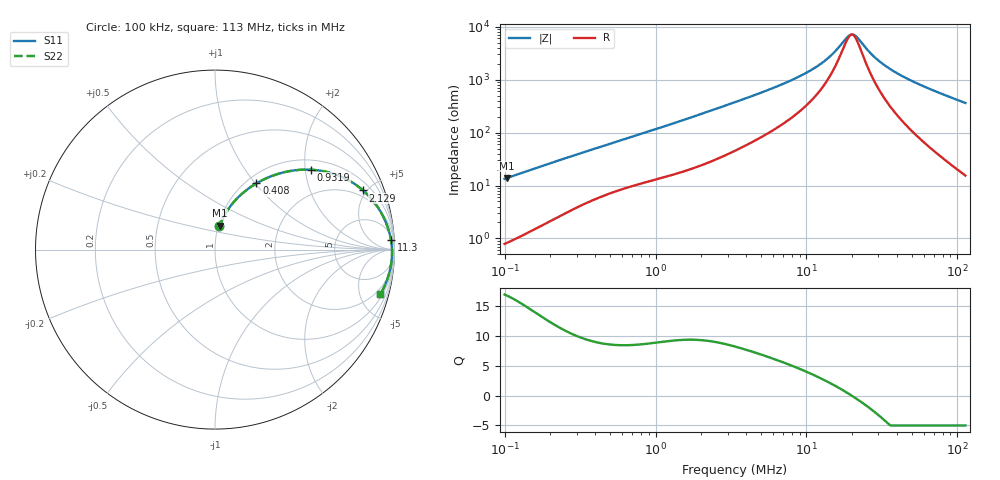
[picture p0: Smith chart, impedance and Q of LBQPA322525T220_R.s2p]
! LBQPA322525T220_R  S-PARAMETER MODEL  ( General Type )
! Model Generated by TAIYO YUDEN Corporation (http://www.ty-top.com)
! Version 1.0
! TAIYO YUDEN Control No. 191025NI43SB-FBB
! Copyright(c) 2019 TAIYO YUDEN CO.,LTD. All Rights Reserved.
! Product Description (link to TY-COMPAS)
! https://ds.yuden.co.jp/TYCOMPAS/or/detail?pn=LBQPA322525T220KR&u=M
! Products Name : Inductors
! Characteristics :
!  Inductance : 22 uH , SRF(min) : 17 MHz , DC Resistance(max) : 0.351 Ohm
!  Rated Current : Saturation :620 mA , Temp Rise : 500 mA (20 degC)
!  Case Size : 3.2 x 2.5 / 0.126 x 0.098 [mm/inch] , Thickness : 2.5 / 0.098 [mm/inch]
!  (Conditions: Temperature = 25 degC , DC Bias Current/Voltage = 0A / 0V)
! External Node Assignments :
!  1  o---GGG---o  2
! GND o---------o GND
! Frequency Range : 0.1MHz  -  113.020708MHz  [ 402 STEP ]
# MHz S RI R 50
! Freq[MHz].  S11 Real  S11 Imag  S21 Real  S21 Imag  S12 Real  S12 Imag  S22 Real  S22 Imag
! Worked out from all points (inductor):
!   401 points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, 100 kHz to 113 MHz, reference 50 ohm
!   read as one part in series: L = 21.1 uH near 103.6 kHz
!   highest Q = 16.8 at 103.6 kHz (marker M1), where L = 21.2 uH
!   self-resonance near 19.95 MHz
!   S11 on the Smith chart (normalised r, x): 100 kHz: 1.02, +0.27; 408 kHz: 1.11, +1.01; 931.9 kHz: 1.24, +2.15; 2.129 MHz: 1.51, +4.74; 11.3 MHz: 10, +32; 113 MHz: 1.31, -7.26
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0.1  0.0249 0.1291  0.9751 -0.1291  0.9751 -0.1291  0.0249 0.1291
0.103578  0.0264 0.1334  0.9736 -0.1334  0.9736 -0.1334  0.0264 0.1334
0.19161  0.0756 0.2277  0.9244 -0.2277  0.9244 -0.2277  0.0756 0.2277
0.324641  0.1702 0.3277  0.8298 -0.3277  0.8298 -0.3277  0.1702 0.3277
0.407973  0.2308 0.3691  0.7692 -0.3691  0.7692 -0.3691  0.2308 0.3691
0.644298  0.386 0.4313  0.614 -0.4313  0.614 -0.4313  0.386 0.4313
0.931918  0.5353 0.445  0.4647 -0.445  0.4647 -0.445  0.5353 0.445
1.053921  0.5862 0.4398  0.4138 -0.4398  0.4138 -0.4398  0.5862 0.4398
1.524399  0.7272 0.3952  0.2728 -0.3952  0.2728 -0.3952  0.7272 0.3952
2.128745  0.8255 0.3293  0.1745 -0.3293  0.1745 -0.3293  0.8255 0.3293
3.421463  0.9116 0.2293  0.0884 -0.2293  0.0884 -0.2293  0.9116 0.2293
6.91079  0.9658 0.1136  0.0342 -0.1136  0.0342 -0.1136  0.9658 0.1136
10.91398  0.9794 0.0594  0.0206 -0.0594  0.0206 -0.0594  0.9794 0.0594
11.30443  0.9801 0.0557  0.0199 -0.0557  0.0199 -0.0557  0.9801 0.0557
14.45804  0.9838 0.0309  0.0162 -0.0309  0.0162 -0.0309  0.9838 0.0309
18.81927  0.9859 0.00559  0.0141 -0.00559  0.0141 -0.00559  0.9859 0.00559
20.18991  0.9863 -0.00113  0.0137 0.00113  0.0137 0.00113  0.9863 -0.00113
21.66037  0.9864 -0.00788  0.0136 0.00788  0.0136 0.00788  0.9864 -0.00788
28.19417  0.9861 -0.034  0.0139 0.034  0.0139 0.034  0.9861 -0.034
35.43129  0.9843 -0.0586  0.0157 0.0586  0.0157 0.0586  0.9843 -0.0586
56.94756  0.9734 -0.1204  0.0266 0.1204  0.0266 0.1204  0.9734 -0.1204
113.0207  0.9205 -0.2501  0.0795 0.2501  0.0795 0.2501  0.9205 -0.2501
